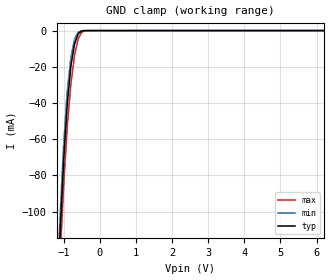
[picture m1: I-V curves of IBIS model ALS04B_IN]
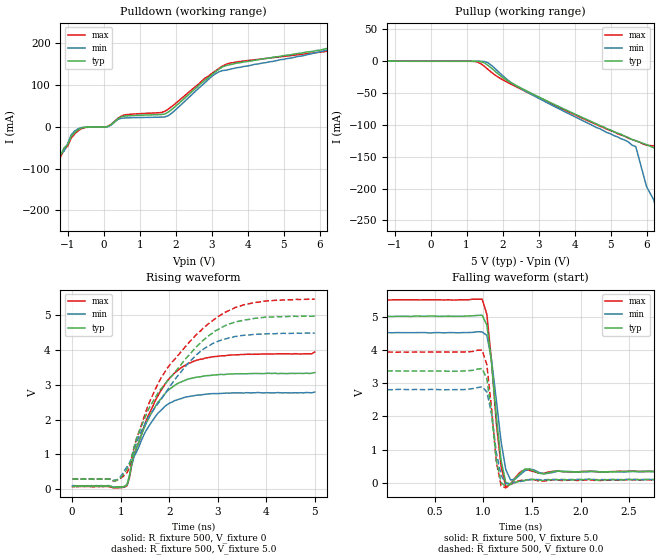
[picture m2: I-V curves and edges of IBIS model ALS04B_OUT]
| TEXAS INSTRUMENTS INCORPORATED
| Standard Linear and Logic Group
| IBIS Model of SN74ALS04B
| HEX INVERTERS
| SOIC 14-pin (D), SOP 14-pin (NS), SSOP 14-pin (DB),PDIP 14-pin (N) Package
[IBIS Ver]   3.2
[Comment Char]  |_char
[File Name]   sn74als04b.ibs
[File Rev]   4.1
[Date]   Sept. 16, 2004
[Source]   Data created from Lab data at TI-SLL.
[Notes]   The following is an IBIS list for the ALS04B.
   - FILE REV HISTORY
   - 4.1 RE-Release IBIS file on 09/23/04
   - Power clamp data deleted as there is no power-clamp diode.
|   - Please contact sllibis@ti.com with questions and
|   comments concerning SLL IBIS models.
[Disclaimer] Property of Texas Instruments Incorporated.  Unauthorized
   reproduction and/or distribution is strictly prohibited.
   This product is protected under copyright law.
   Created 2000, (C) Copyright 2000, Texas Instruments Inc.,
   All Rights Reserved.
   UNLESS THERE IS A SIGNED, WRITTEN AGREEMENT TO THE
   CONTRARY, TEXAS INSTRUMENTS () IS PROVIDING THE IBIS
   MODELS  AND WITHOUT ANY WARRANTY, EXPRESSED OR
   IMPLIED.  TI assumes no liability for:
   1) the accuracy of the IBIS models provided to your
   company;
   2) the proper functioning of these IBIS Models in your
   design or for any resulting applications; or
   3) infringement of patents, copyrights or intellectual
   property rights resulting from your use of these IBIS
   models.
   TI provides IBIS Models as a service to our customers.
   You and your company shall not distribute, sell or give
   these models to anyone else without prior written
   permission from TI.
   TI reserves the right to make changes to our products or
   to discontinue any semiconductor product or service
   without notice, and advises our customers to obtain the
   latest version of relevant information to verify, before
   placing orders, that the information being relied on is
   current.
   Please be aware that your receipt and use of the IBIS
   information provided shall serve as acceptance of these
   terms and conditions.  If you do not accept these terms,
   you should return or destroy the IBIS models and any
   other accompanying information immediately.
|   Component ALS04B_D
[Component]   ALS04B_D
[Manufacturer]  Texas Instruments, Inc.
[Package]
|   typ   min   max
R_pkg   0.031   0.028   0.034
L_pkg   3.109nH   2.462nH   3.889nH
C_pkg   0.473pF   0.363pF   0.628pF
[Pin]   signal_name   model_name   R_pin   L_pin   C_pin
1   1A   ALS04B_IN   0.033   3.854nH   0.622pF
2   1Y   ALS04B_OUT   0.032   3.188nH   0.473pF
3   2A   ALS04B_IN   0.028   2.462nH   0.377pF
4   2Y   ALS04B_OUT   0.031   2.596nH   0.363pF
5   3A   ALS04B_IN   0.028   2.521nH   0.372pF
6   3Y   ALS04B_OUT   0.034   3.250nH   0.476pF
7   GND   GND   0.034   3.889nH   0.628pF
8   4Y   ALS04B_OUT   0.034   3.889nH   0.628pF
9   4A   ALS04B_IN   0.034   3.250nH   0.476pF
10   5Y   ALS04B_OUT   0.028   2.521nH   0.372pF
11   5A   ALS04B_IN   0.031   2.596nH   0.364pF
12   6Y   ALS04B_OUT   0.028   2.462nH   0.377pF
13   6A   ALS04B_IN   0.032   3.188nH   0.473pF
14   VCC   POWER   0.033   3.854nH   0.622pF
|   Component ALS04B_NS
[Component]   ALS04B_NS
[Manufacturer]  Texas Instruments, Inc
[Package]
|   typ   min   max
R_pkg   0.045   0.039   0.054
L_pkg   3.796nH   2.561nH   4.952nH
C_pkg   0.528pF   0.288pF   0.710pF
[Pin]   signal_name   model_name   R_pin   L_pin   C_pin
1   1A   ALS04B_IN   0.047   4.867nH   0.706pF
2   1Y   ALS04B_OUT   0.051   4.083nH   0.592pF
3   2A   ALS04B_IN   0.041   2.915nH   0.376pF
4   2Y   ALS04B_OUT   0.039   2.561nH   0.288pF
5   3A   ALS04B_IN   0.041   3.101nH   0.430pF
6   3Y   ALS04B_OUT   0.047   4.047nH   0.589pF
7   GND   GND   0.051   4.909nH   0.700pF
8   4Y   ALS04B_OUT   0.045   4.784nH   0.694pF
9   4A   ALS04B_IN   0.054   4.176nH   0.597pF
10   5Y   ALS04B_OUT   0.039   3.287nH   0.449pF
11   5A   ALS04B_IN   0.039   2.586nH   0.294pF
12   6Y   ALS04B_OUT   0.040   2.802nH   0.371pF
13   6A   ALS04B_IN   0.049   4.080nH   0.593pF
14   VCC   POWER   0.052   4.952nH   0.710pF
|   Component ALS04B_DB
[Component]   ALS04B_DB
[Manufacturer]  Texas Instruments, Inc.
[Package]
|   typ   min   max
R_pkg   0.044   0.041   0.046
L_pkg   3.551nH   3.258nH   3.927nH
C_pkg   0.402pF   0.360pF   0.421pF
[Pin]   signal_name   model_name   R_pin   L_pin   C_pin
1   1A   ALS04B_IN   0.046   3.927nH   0.408pF
2   1Y   ALS04B_OUT   0.044   3.587nH   0.421pF
3   2A   ALS04B_IN   0.041   3.289nH   0.398pF
4   2Y   ALS04B_OUT   0.042   3.258nH   0.360pF
5   3A   ALS04B_IN   0.041   3.286nH   0.403pF
6   3Y   ALS04B_OUT   0.044   3.586nH   0.421pF
7   GND   GND   0.046   3.927nH   0.408pF
8   4Y   ALS04B_OUT   0.046   3.927nH   0.408pF
9   4A   ALS04B_IN   0.044   3.586nH   0.421pF
10   5Y   ALS04B_OUT   0.041   3.286nH   0.403pF
11   5A   ALS04B_IN   0.043   3.258nH   0.360pF
12   6Y   ALS04B_OUT   0.041   3.289nH   0.398pF
13   6A   ALS04B_IN   0.044   3.587nH   0.421pF
14   VCC   POWER   0.046   3.927nH   0.408pF
|   Component ALS04B_N
[Component]   ALS04B_N
[Manufacturer]   Texas Instruments, Inc.
[Package]
|   typ   min   max
R_pkg   4.500e-02   3.700e-02   6.300e-02
L_pkg   5.407e-09   3.922e-09   6.942e-09
C_pkg   3.890e-13   2.050e-13   6.040e-13
[Pin]   signal_name   model_name   R_pin   L_pin   C_pin
1   1A   ALS04B_IN   6.300e-02   6.942e-09   6.040e-13
2   1Y   ALS04B_OUT   3.700e-02   6.200e-09   4.060e-13
3   2A   ALS04B_IN   4.200e-02   4.389e-09   3.220e-13
4   2Y   ALS04B_OUT   3.800e-02   3.922e-09   2.050e-13
5   3A   ALS04B_IN   3.900e-02   4.301e-09   2.980e-13
6   3Y   ALS04B_OUT   3.800e-02   5.329e-09   3.560e-13
7   GND   GND   5.300e-02   6.510e-09   5.440e-13
8   4Y   ALS04B_OUT   5.300e-02   6.437e-09   5.390e-13
9   4A   ALS04B_IN   3.900e-02   5.352e-09   3.470e-13
10   5Y   ALS04B_OUT   4.200e-02   4.473e-09   2.970e-13
11   5A   ALS04B_IN   4.400e-02   4.326e-09   2.250e-13
12   6Y   ALS04B_OUT   4.200e-02   4.295e-09   2.800e-13
13   6A   ALS04B_IN   4.200e-02   6.318e-09   4.180e-13
14   VCC   POWER   6.100e-02   6.900e-09   6.030e-13
| Models and submodels in the file (2): ALS04B_IN (Input), ALS04B_OUT (Output)
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|   Model ALS04B_IN
[Model]   ALS04B_IN
Model_type  Input
Polarity   Non-Inverting
Vinl = 0.8
Vinh = 2.0
| variable   typ   min   max
C_comp   1.24pf   0.94pf   1.54pf
[Temperature Range]   25   0   70
[Voltage Range]   5.0   4.5   5.5
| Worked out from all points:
|   GND clamp passes 1 mA (typ) near -0.55 V on its own axis
[GND Clamp]
|   Voltage   I(typ)   I(min)   I(max)
-5V       -1.11A     -1.55A     -1.01A
-1.2V     -159mA     -150mA     -170mA
-1.1V     -112mA     -102mA     -125mA
-1V       -71.1mA    -62mA      -84.9mA
-900mV    -40mA      -32.6mA    -52.4mA
-800mV    -19.3mA    -14.4mA    -29mA
-700mV    -7.33mA    -4.66mA    -13.6mA
-600mV    -1.78mA    -856uA     -4.54mA
-500mV    -164uA     -46.2uA    -872uA
-400mV    -12.1uA    -7.75uA    -69uA
-300mV    -6.77uA    -6.6uA     -8.67uA
10V       2.8nA      6.54pA     97.2pA
|   Model ALS04B_OUT
[Model]   ALS04B_OUT
Model_type  Output
Polarity   Inverting
Vmeas = 2.50v
Cref = 15pf
| variable   typ   min   max
C_comp   4.62pf   3.47pf   5.77pf
[Temperature Range]   25   0   70
[Voltage Range]   5.0   4.5   5.5
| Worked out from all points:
|   slope of the pulldown table from 0 to 0.75 V, typ, clamps not added: 27.5 ohm
|   rising waveform, R_fixture 500, V_fixture 0: 20-80 % time 663ps typ, 602ps min, 743ps max; typ from 0.085 V to 3.35 V
|   falling waveform, R_fixture 500, V_fixture 5.0: 20-80 % time 95.8ps typ, 101ps min, 92.8ps max; typ from 5.02 V to 0.345 V
|   rising waveform, R_fixture 500, V_fixture 5.0: 20-80 % time 1.24ns typ, 1.13ns min, 1.25ns max; typ from 0.29 V to 4.96 V
|   falling waveform, R_fixture 500, V_fixture 0.0: 20-80 % time 75.5ps typ, 81.7ps min, 76.4ps max; typ from 3.37 V to 0.092 V
[Pulldown]
|   Voltage   I(typ)   I(min)   I(max)
-5V       -948mA     -986mA     -905mA
-2V       -250mA     -254mA     -245mA
-1.9V     -227mA     -230mA     -223mA
-1.2V     -68.4mA    -63.8mA    -72.4mA
-800mV    -12.8mA    -9.46mA    -16.4mA
-500mV    -671uA     -475uA     -1.19mA
100mV     473uA      111uA      880uA
600mV     26.2mA     21.5mA     29.2mA
1.8V      35.8mA     27.2mA     42.9mA
3.3V      144mA      135mA      146mA
6.8V      199mA      199mA      190mA
10V       228mA      232mA      250mA
[Pullup]
|   Voltage   I(typ)   I(min)   I(max)
-5V       30.43mA    49.66mA    9.951mA
-1.7V     2.69mA     2.08mA     1.895mA
1.3V      -105uA     -27.4uA    -1.18mA
5.7V      -125mA     -134mA     -125mA
6V        -131mA     -197mA     -132mA
6.3V      -138mA     -239mA     -134mA
6.4V      -160mA     -260mA     -136mA
6.8V      -249mA     -344mA     -145mA
6.9V      -271mA     -365mA     -168mA
7V        -293mA     -386mA     -191mA
7.6V      -425mA     -512mA     -331mA
10V       -953mA     -1.016A    -883mA
[Ramp]
| variable   typ   min   max
dV/dt_r   1.94E+00/6.69E-09   1.60E+00/6.11E-09   2.28E+00/7.34E-09
dV/dt_f   2.81E+00/9.00E-10   2.51E+00/1.00E-09   3.10E+00/8.90E-10
R_load = 500
[Rising Waveform]
R_fixture = 500
V_fixture = 0
C_fixture = 0pf
L_fixture = 0nH
|   Time   V(typ)   V(min)   V(max)
9.766ps   84.66mV    105.1mV    72.41mV
839.8ps   53.56mV    68.25mV    48.25mV
1.133ns   137.3mV    127.6mV    109mV
1.182ns   397.8mV    373.6mV    330.6mV
1.279ns   1.026V     943.1mV    993.1mV
1.621ns   2.149V     1.896V     2.258V
1.963ns   2.817V     2.43V      3.11V
2.354ns   3.143V     2.649V     3.574V
3.066ns   3.295V     2.749V     3.825V
5ns       3.348V     2.788V     3.938V
[Falling Waveform]
R_fixture = 500
V_fixture = 5.0
V_fixture_min = 4.5
V_fixture_max = 5.5
C_fixture = 0pf
L_fixture = 0nH
|   Time   V(typ)   V(min)   V(max)
9.766ps   5.019V     4.528V     5.51V
986.3ps   5.05V      4.548V     5.536V
1.035ns   4.757V     4.443V     5.079V
1.084ns   3.588V     3.689V     3.643V
1.133ns   1.979V     2.479V     1.787V
1.182ns   660.9mV    1.228V     485mV
1.23ns    10.44mV    397mV      -126.3mV
1.279ns   -46.75mV   82.78mV    -38.62mV
1.426ns   409.4mV    360.3mV    396.4mV
5ns       345.1mV    338.9mV    346.5mV
[Rising Waveform]
R_fixture = 500
V_fixture = 5.0
V_fixture_min = 4.5
V_fixture_max = 5.5
C_fixture = 0pf
L_fixture = 0nH
|   Time   V(typ)   V(min)   V(max)
9.766ps   290.3mV    295.4mV    295.9mV
888.7ps   245.6mV    266.2mV    243.1mV
1.133ns   577.5mV    650.1mV    480.4mV
1.328ns   1.455V     1.342V     1.453V
1.523ns   2.13V      1.925V     2.233V
1.816ns   2.855V     2.54V      3.15V
2.402ns   3.838V     3.632V     4.197V
2.949ns   4.541V     4.212V     4.891V
3.711ns   4.888V     4.435V     5.34V
5ns       4.963V     4.478V     5.451V
[Falling Waveform]
R_fixture = 500
V_fixture = 0.0
V_fixture_min = 0.0
V_fixture_max = 0.0
C_fixture = 0pf
L_fixture = 0nH
|   Time   V(typ)   V(min)   V(max)
9.766ps   3.366V     2.805V     3.941V
986.3ps   3.442V     2.894V     3.997V
1.035ns   3.135V     2.737V     3.559V
1.084ns   2.09V      2.072V     2.227V
1.133ns   670mV      899.7mV    616.7mV
1.182ns   4.032mV    221.4mV    -93mV
1.23ns    -108.6mV   -28.62mV   -154.6mV
1.328ns   10.75mV    6.376mV    37.94mV
1.475ns   99.35mV    94.03mV    94.97mV
5ns       92.47mV    102.3mV    84.5mV
